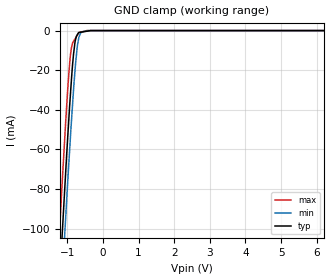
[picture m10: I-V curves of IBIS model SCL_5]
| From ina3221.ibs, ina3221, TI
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[Model]   SCL_5
Model_type   Input
Vinl = 1.5   |min, GND -0.5 V
Vinh = 3.5   |max. V+ 6 V
|   typ   min   max
|   (nom PVT)   (Fast PVT)   (slow PVT)
C_comp   1.406E-12   1.362E-12   1.406E-12
| Where   nom PVT is  Nominal Process, 3.3V, 25C
|   Fast PVT is Strong Process, 3.6V, -40C
|   Slow PVT is Weak Process, 3.0V, 85C
|C_comp - from L-C Tank method, L = 1nH, peak frequency
[Model Spec]
| variable   typ   min   max
Vinl   1.5   1.35   1.65
Vinh   3.5   3.15   3.85
|Vinl = 0.3 x V+, Vinh = 0.7 x V+
[Voltage Range]   5   4.5   5.5
|Ambient Temperature Range   27   85   -40
[Temperature Range]   30   88   -40
[Power Clamp Reference]   5   4.5   5.5
[GND Clamp Reference]   0   0   0
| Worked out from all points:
|   GND clamp passes 1 mA (typ) near -0.68 V on its own axis
[GND Clamp]
|   Voltage   I(typ)   I(min)   I(max)
-5V       -1.44A     -1.448A    -1.433A
-1.243V   -135mA     -157.3mA   -109.8mA
-1.129V   -98.53mA   -121.2mA   -72.44mA
-1.045V   -71.39mA   -94.31mA   -45.96mA
-981.9mV  -52.2mA    -74.56mA   -28.02mA
-910.1mV  -31.87mA   -53.38mA   -12.17mA
-850.4mV  -17.01mA   -36.99mA   -6.279mA
-785.7mV  -6.169mA   -20.79mA   -4.288mA
-682.8mV  -1.011mA   -4.257mA   -1.256mA
-610.6mV  -797.1uA   -790.4uA   -712.4uA
-423.9mV  -244.3uA   -4.682uA   -4.099uA
9.985V    0A         0A         0A
[POWER Clamp]
|   SCR cell for ESD function. Effects occurr above VDD x 2
|   Voltage   I(typ)   I(min)   I(max)
-5V       0A         0A         0A
0V        0A         0A         0A
10V       0A         0A         0A
